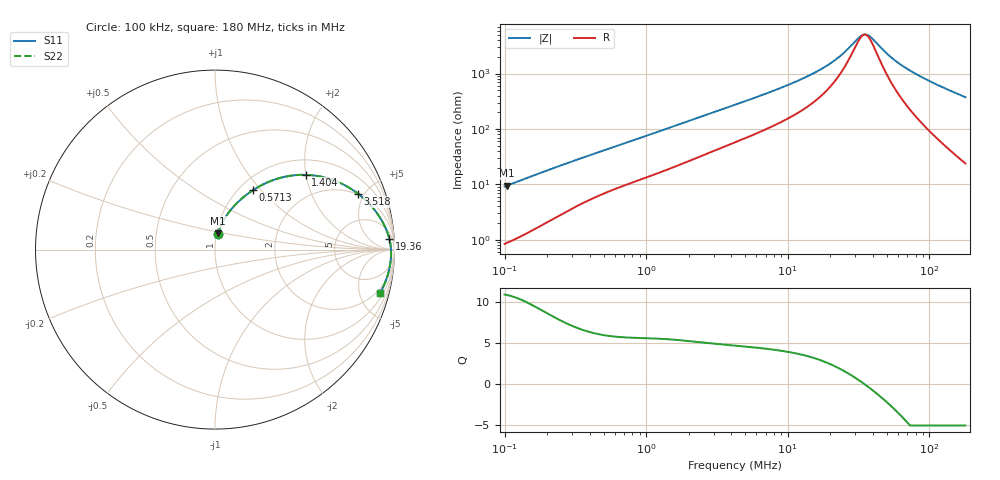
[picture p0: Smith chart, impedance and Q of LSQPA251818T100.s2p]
! LSQPA251818T100  S-PARAMETER MODEL  ( General Type )
! Model Generated by TAIYO YUDEN Corporation (http://www.ty-top.com)
! Version 3.0
! TAIYO YUDEN Control No. 160907NF25SB-FAC
! Copyright(c) 2007 TAIYO YUDEN CO.,LTD. All Rights Reserved.
! Product Description (link to TY-COMPAS)
! https://ds.yuden.co.jp/TYCOMPAS/or/detail?pn=LSQPA251818T100K&u=M
! Products Name : Inductors
! Characteristics :
!  Inductance : 10 uH , SRF(min) : 30 MHz , DC Resistance(max) : 0.468 Ohm
!  Rated Current : Saturation :480 mA , Temp Rise : 680 mA (40 degC)
!  Case Size : 2.5 x 1.8 / 0.098 x 0.071 [mm/inch] , Thickness : 1.8 / 0.071 [mm/inch]
!  (Conditions: Temperature = 25 degC , DC Bias Current/Voltage = 0A / 0V)
! External Node Assignments :
!  1  o---GGG---o  2
! GND o---------o GND
! Frequency Range : 0.1MHz  -  180.004543MHz  [ 402 STEP ]
# MHz S RI R 50
! Freq[MHz].  S11 Real  S11 Imag  S21 Real  S21 Imag  S12 Real  S12 Imag  S22 Real  S22 Imag
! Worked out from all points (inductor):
!   401 points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, 100 kHz to 180 MHz, reference 50 ohm
!   read as one part in series: L = 14.4 uH near 103.8 kHz
!   highest Q = 10.8 at 103.8 kHz (marker M1), where L = 14.4 uH
!   self-resonance near 34.89 MHz
!   S11 on the Smith chart (normalised r, x): 100 kHz: 1.02, +0.18; 571.3 kHz: 1.16, +0.90; 1.404 MHz: 1.37, +1.99; 3.518 MHz: 1.94, +4.51; 19.36 MHz: 12, +27; 180 MHz: 1.48, -7.48
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0.1  0.0163 0.0886  0.9837 -0.0886  0.9837 -0.0886  0.0163 0.0886
0.103819  0.0172 0.0917  0.9828 -0.0917  0.9828 -0.0917  0.0172 0.0917
0.203822  0.0503 0.1674  0.9497 -0.1674  0.9497 -0.1674  0.0503 0.1674
0.350962  0.1135 0.2504  0.8865 -0.2504  0.8865 -0.2504  0.1135 0.2504
0.571286  0.2105 0.3304  0.7895 -0.3304  0.7895 -0.3304  0.2105 0.3304
1.231743  0.4562 0.4154  0.5438 -0.4154  0.5438 -0.4154  0.4562 0.4154
1.404389  0.5059 0.4165  0.4941 -0.4165  0.4941 -0.4165  0.5059 0.4165
2.286024  0.6796 0.379  0.3204 -0.379  0.3204 -0.379  0.6796 0.379
3.517707  0.7969 0.3113  0.2031 -0.3113  0.2031 -0.3113  0.7969 0.3113
4.322947  0.8393 0.2753  0.1607 -0.2753  0.1607 -0.2753  0.8393 0.2753
8.811135  0.9307 0.1593  0.0693 -0.1593  0.0693 -0.1593  0.9307 0.1593
14.89024  0.9623 0.0907  0.0377 -0.0907  0.0377 -0.0907  0.9623 0.0907
19.35694  0.9713 0.061  0.0287 -0.061  0.0287 -0.061  0.9713 0.061
24.23791  0.9765 0.0372  0.0235 -0.0372  0.0235 -0.0372  0.9765 0.0372
32.10467  0.9801 0.00845  0.0199 -0.00845  0.0199 -0.00845  0.9801 0.00845
34.60359  0.9806 0.000834  0.0194 -0.000834  0.0194 -0.000834  0.9806 0.000834
36.6046  0.9809 -0.0049  0.0191 0.0049  0.0191 0.0049  0.9809 -0.0049
38.72134  0.9811 -0.0107  0.0189 0.0107  0.0189 0.0107  0.9811 -0.0107
52.25907  0.9805 -0.0426  0.0195 0.0426  0.0195 0.0426  0.9805 -0.0426
65.43652  0.9779 -0.069  0.0221 0.069  0.0221 0.069  0.9779 -0.069
85.06583  0.9721 -0.1038  0.0279 0.1038  0.0279 0.1038  0.9721 -0.1038
180.0045  0.9202 -0.241  0.0798 0.241  0.0798 0.241  0.9202 -0.241
